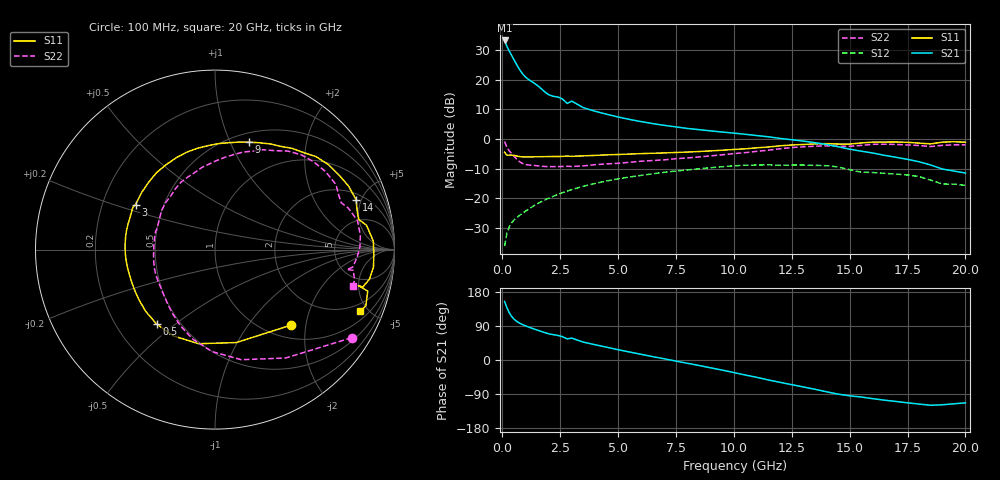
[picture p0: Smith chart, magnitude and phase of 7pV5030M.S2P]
! Infineon Technologies  Discrete & RF Semiconductors
! bfp620
! VCE = 0.50 V,  IC =  30 mA
! Common Emitter S-Parameters:  Sep 2002
# GHz  S  MA  R  50
!  f  S11  S21  S12  S22
! GHz  MAG  ANG  MAG  ANG  MAG  ANG  MAG  ANG
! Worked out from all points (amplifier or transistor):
!   59 points, 100 MHz to 20 GHz, reference 50 ohm
!   highest |S21| = 33.2 dB at 100 MHz (marker M1)
!   |S21| within 3 dB of that: start of sweep to 263.6 MHz
!   unconditionally stable (mu >= 1): 2.681 GHz to 2.918 GHz; 3.188 GHz to 10.15 GHz; 17.11 GHz to end of sweep
!   at 1 GHz: K = 0.81, MSG = 22.6 dB, |S12| = -24.4 dB
!   at 5.5 GHz: K = 1.05, MAG = 8.3 dB, |S12| = -12.8 dB
!   at 20 GHz: K = 1.66, MAG = -2.7 dB, |S12| = -15.6 dB
!   S11 on the Smith chart (normalised r, x): 100 MHz: 1.26, -1.65; 500 MHz: 0.37, -0.43; 3 GHz: 0.35, +0.23; 9 GHz: 0.60, +1.18; 14 GHz: 2.47, +4.51; 20 GHz: 1.47, -4.45
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0.1  0.597 -44.8  45.57 154.3  0.0156 68.9  0.9062 -32.8
0.2  0.5314 -77.1  36.2 138.0  0.0258 57.8  0.721 -56.9
0.3  0.5322 -99.9  30.2 124.9  0.0331 53.5  0.6307 -76.6
0.4  0.5339 -115.8  25.61 115.2  0.0385 51.1  0.5681 -91.8
0.5  0.5273 -128.1  21.74 108.2  0.0428 49.8  0.5134 -104.1
0.6  0.5171 -138.2  18.47 102.9  0.0464 49.2  0.4657 -114.5
0.7  0.5078 -146.6  15.79 98.8  0.0499 49.0  0.4276 -123.6
0.9  0.498 -159.0  12.16 92.7  0.0569 49.4  0.3821 -138.2
1.1  0.4971 -167.0  10.25 87.8  0.0644 49.9  0.3652 -148.1
1.5  0.5005 -178.7  8.043 79.2  0.0801 49.9  0.3532 -162.6
2  0.5043 167.7  5.571 69.3  0.0999 47.9  0.3415 -179.7
2.6  0.5083 157.2  4.708 61.5  0.1241 44.1  0.3434 168.6
2.8  0.5147 152.6  3.954 55.7  0.1319 42.5  0.3462 162.5
3  0.5088 150.5  4.332 57.7  0.1401 40.9  0.3435 161.9
3.5  0.5183 141.7  3.36 47.2  0.1594 36.3  0.3512 152.2
7  0.5807 93.6  1.692 3.1  0.2737 2.1  0.4443 104.5
9  0.6285 72.3  1.365 -20.7  0.3274 -19.0  0.5181 83.7
10.5  0.6818 57.5  1.196 -39.8  0.3606 -37.3  0.5875 69.0
13.5  0.8238 25.5  0.864 -77.2  0.3583 -73.0  0.7538 35.2
14  0.8337 19.5  0.807 -83.8  0.3548 -80.0  0.7652 28.4
17  0.8883 -6.3  0.49 -109.4  0.255 -104.2  0.8073 0.9
20  0.8794 -23.0  0.266 -113.1  0.1652 -115.6  0.7945 -14.7
